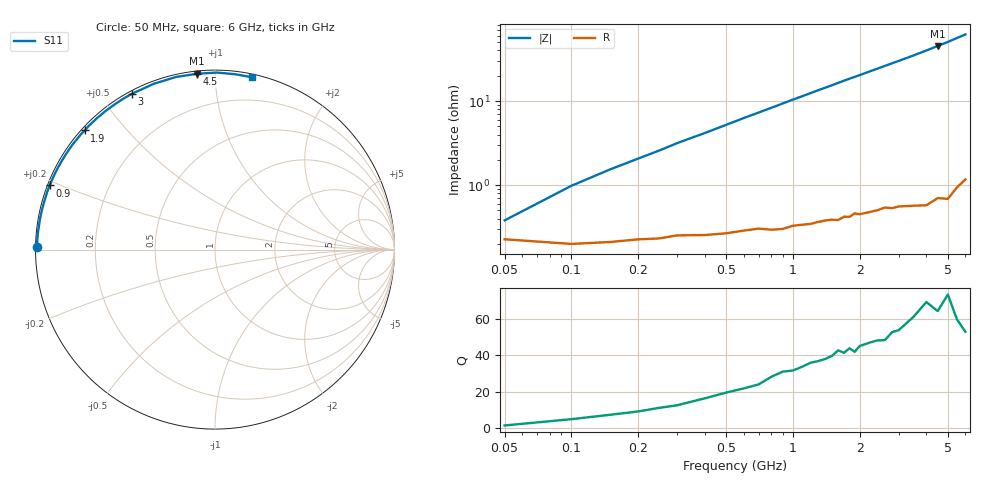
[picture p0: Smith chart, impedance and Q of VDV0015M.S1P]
! Infineon Technologies  Discrete & RF Semiconductors
! BBY 55-03
! Si Tuning Diode in SOD323
! VR =
! S-Parameters:  June  1999
# GHz  S  MA  R  50
!  f  S11
! GHz  MAG  ANG
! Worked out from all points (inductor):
!   34 points, 50 MHz to 6 GHz, reference 50 ohm
!   read as one part to ground: L = 1.62 nH near 100 MHz
!   highest Q = 69.5 at 4.5 GHz (marker M1), where L = 1.6 nH
!   S11 on the Smith chart (normalised r, x): 50 MHz: 0.00, +0.01; 900 MHz: 0.01, +0.19; 1.9 GHz: 0.01, +0.39; 3 GHz: 0.01, +0.60; 4.5 GHz: 0.01, +0.90; 6 GHz: 0.02, +1.24
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0.05  0.991 179.3
0.1  0.992 177.8
0.15  0.9916 176.5
0.25  0.9908 174.1
0.3  0.99 172.8
0.4  0.9899 170.5
0.5  0.9895 168.1
0.6  0.9887 165.7
0.8  0.9886 161.1
0.9  0.9884 158.8
1  0.9875 156.5
1.1  0.9872 154.3
1.3  0.9865 149.9
1.6  0.9862 143.6
1.8  0.9853 139.5
1.9  0.9841 137.6
2  0.9847 135.7
2.2  0.9843 131.9
2.4  0.9839 128.3
2.6  0.9832 124.7
2.8  0.984 121.3
3  0.9838 118.0
3.5  0.9848 110.2
4  0.9861 102.7
4.5  0.9847 95.8
5  0.9865 89.4
5.5  0.9836 83.2
6  0.9818 77.8
